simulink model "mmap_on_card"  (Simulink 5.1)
settings: Solver=ode45  StartTime=0.0  StopTime=100.0  RelTol=1e-3
libraries: ADlibrary x1

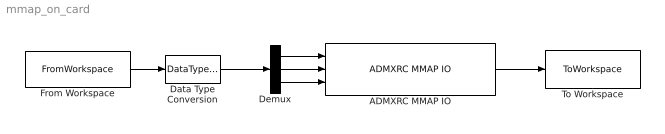
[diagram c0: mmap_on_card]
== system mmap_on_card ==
  ADMXRC MMAP IO : ADlibrary/Hardware in the Loop/ADMXRC MMAP IO  filename=e:/tmp1/mmap.bit  clock_freq=33  mclk_freq=40  index=0
  Data Type Conversion : DataTypeConversion  DataType=uint32
  Demux : Demux  Outputs=3
  From Workspace : FromWorkspace  InitFcn=init_mmap_program  VariableName=mmap_program  SampleTime=0
  To Workspace : ToWorkspace  VariableName=mmap_output  SampleTime=-1  SaveFormat=Structure
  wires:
  From Workspace/1 -> Data Type Conversion/1
  Demux/1 -> ADMXRC MMAP IO/1
  Demux/2 -> ADMXRC MMAP IO/2
  Demux/3 -> ADMXRC MMAP IO/3
  ADMXRC MMAP IO/1 -> To Workspace/1
  Data Type Conversion/1 -> Demux/1
